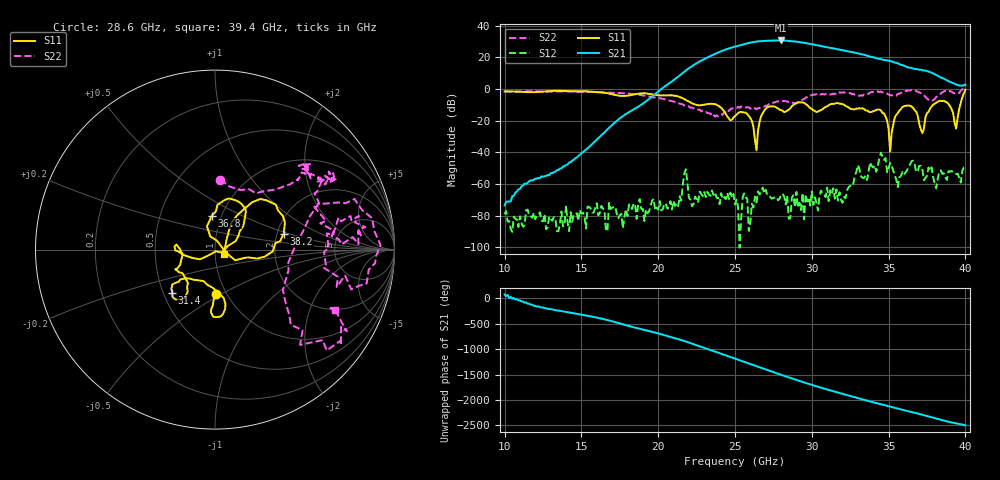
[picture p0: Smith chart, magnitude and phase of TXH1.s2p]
!Keysight Technologies,M9808A,MY58100618,A.14.70.03
!Date: Monday, February 27, 2023 13:18:08
!Correction: S11(C  2-Port  )
!S21(C  2-Port  )
!S12(C  2-Port  )
!S22(C  2-Port  )
!S2P File: Measurements: S11, S21, S12, S22:
# Hz S  RI  R 50
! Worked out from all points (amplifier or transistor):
!   301 points, 10 GHz to 40 GHz, reference 50 ohm
!   highest |S21| = 30.6 dB at 28 GHz (marker M1)
!   |S21| within 3 dB of that: 25.33 GHz to 30.33 GHz (5.008 GHz wide, 18 % of centre)
!   unconditionally stable (mu >= 1): start of sweep to 39.81 GHz
!   at 15 GHz: K = 49839.37, MAG = -31.1 dB, |S12| = -78.7 dB
!   at 25 GHz: K = 94.90, MAG = 27.1 dB, |S12| = -73.1 dB
!   at 40 GHz: K = -12.27, MSG = 26.0 dB, |S12| = -49.6 dB
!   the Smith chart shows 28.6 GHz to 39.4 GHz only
!   S11 on the Smith chart (normalised r, x): 28.6 GHz: 0.89, -0.47; 31.4 GHz: 0.56, -0.30; 36.8 GHz: 0.90, +0.35; 38.2 GHz: 2.18, +0.46; 39.4 GHz: 1.10, -0.06
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1e10  0.7437 0.3574  7.51e-05 0.000197  -0.000107 2.42e-05  -0.0334 0.8563
1.5e10  0.6364 -0.556  0.00734 0.00529  8.82e-05 -7.56e-05  0.7368 0.3013
2e10  -0.12 -0.6225  0.7386 0.3751  -7.87e-05 0.000132  0.245 -0.4574
2.25e10  -0.2886 -0.1186  -5.866 2.779  0.000327 6.84e-05  -0.0878 -0.2152
2.34e10  -0.338 -0.0284  5.38 9.498  0.000266 0.000323  -0.1137 -0.1222
2.42e10  -0.2144 -0.0686  14.83 -6.42  0.000231 -0.000235  -0.1502 -0.0193
2.5e10  -0.0725 0.1199  -7.04 -20.58  -0.000214 -5.63e-05  -0.2521 0.0615
2.58e10  -0.0764 0.1428  -26.79 6.374  0.000126 0.000316  -0.2454 0.0986
2.66e10  0.0571 -0.071  5.41 31.86  0.000209 0.000415  -0.1339 0.2106
2.73e10  0.2502 -0.1302  33.05 3.784  0.000334 0.000189  -0.0473 0.3378
2.8e10  0.1755 -0.1251  14 -31.04  -0.000339 -0.000306  -0.0057 0.4255
2.86e10  0.00552 -0.2468  -19.68 -26.04  -2.11e-05 7.82e-05  0.028 0.3878
2.92e10  0.00301 -0.3765  -30 3.288  -0.000161 0.000197  0.2289 0.313
3e10  0.0105 -0.2319  -3.075 25.72  0.000403 0.000413  0.4831 0.4301
3.07e10  -0.163 -0.1593  18.7 12.06  -0.000476 8.84e-05  0.5102 0.4817
3.14e10  -0.2386 -0.2392  16.92 -9.023  -0.0002 -0.000701  0.59 0.3974
3.3e10  -0.2075 -0.1192  -12.82 -4.003  -0.00374 0.00116  0.5799 0.2582
3.5e10  -0.0422 -0.0356  6.131 4.872  0.00116 -0.00292  0.6585 0.0829
3.68e10  -0.0171 0.1899  -0.5437 -4.235  0.000443 0.0023  0.8186 0.2215
3.82e10  0.3834 0.0895  -2.146 1.451  0.00106 -0.00103  0.4222 -0.419
3.94e10  0.0491 -0.0263  0.6649 1.207  -0.00205 0.000116  0.6703 -0.3373
4e10  0.4714 -0.8254  1.253 0.4751  -0.00333 -3.77e-05  1.096 -0.9307
